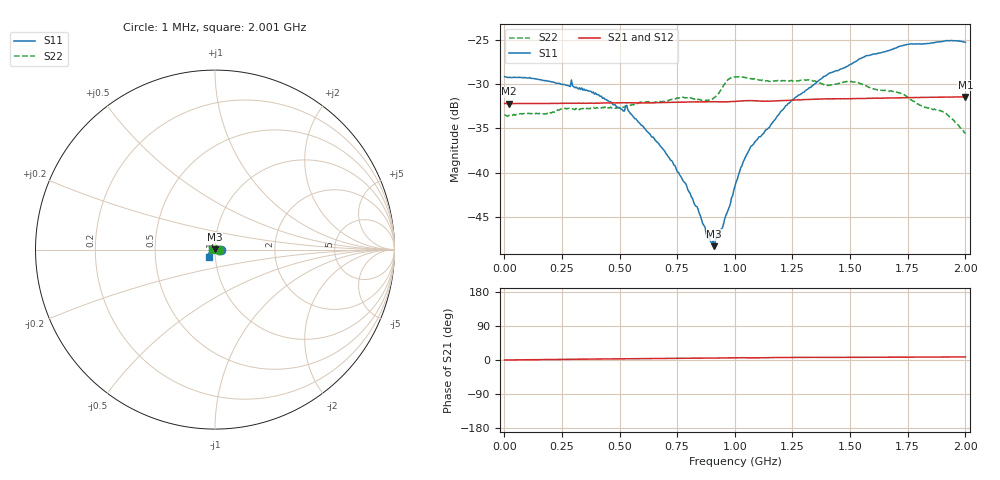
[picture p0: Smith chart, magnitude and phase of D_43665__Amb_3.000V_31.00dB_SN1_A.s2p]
! device id: 43665_
! dir: \\malibu\benchdata\1_engineers\tn_data\43665_75ohm\new\sparar\43665_\amb\3p000v\31p00db
! Serial: 1
! Insertion: A
! Temp: Amb
! VDD: 3.000V
! Attenuation Step: 31.00dB
! IDD: 1.445651e+00mA
! FILE NAME
! DATE 03-27-2009 08:42:13
! CORRECTED  DATA
#  Hz  S  RI  R  75
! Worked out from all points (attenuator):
!   401 points, 1 MHz to 2.001 GHz, reference 75 ohm
!   highest |S21| = -31.44 dB at 2.001 GHz (marker M1); lowest = -32.2 dB at 21 MHz (marker M2)
!   lowest |S11| = -48.3 dB at 911 MHz (marker M3), VSWR 1.01, Z = 74.6 + j0.442 ohm
!   |S11| at or under -10 dB: start of sweep to end of sweep
!   |S22| runs from -35.6 to -29.2 dB; largest |S21 - S12| = 0.00022
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1000000  0.0348 -0.000333  0.0246 4.37e-05  0.0248 -8.65e-05  0.0212 -0.000164
2.1e7  0.0345 0.000212  0.0245 5.04e-05  0.0245 5.75e-05  0.021 0.0012
3.36e8  0.0295 0.00583  0.0246 0.000938  0.0247 0.000944  0.0125 0.0193
5.36e8  0.0212 0.00762  0.0248 0.0014  0.0248 0.00141  0.00159 0.0236
6.71e8  0.0126 0.00719  0.0248 0.00181  0.0248 0.00183  -0.00699 0.024
7.81e8  0.0064 0.00607  0.0249 0.00205  0.0249 0.00209  -0.014 0.0226
8.41e8  0.00266 0.00558  0.025 0.00214  0.025 0.00218  -0.0172 0.0194
8.86e8  -0.00106 0.00431  0.025 0.0022  0.025 0.00222  -0.0197 0.0164
9.11e8  -0.00245 0.00296  0.025 0.00224  0.025 0.00232  -0.0219 0.0149
9.41e8  -0.0043 0.00211  0.025 0.00234  0.025 0.00239  -0.0263 0.0135
9.71e8  -0.00592 0.00164  0.025 0.00246  0.025 0.00251  -0.03 0.0152
1.001e9  -0.00827 0.00141  0.0251 0.00259  0.0251 0.00263  -0.0306 0.0164
1.036e9  -0.0114 0.000566  0.0253 0.00267  0.0253 0.00266  -0.031 0.0154
1.076e9  -0.0142 -0.00141  0.0254 0.00251  0.0254 0.00253  -0.0307 0.0138
1.226e9  -0.023 -0.00702  0.0254 0.00302  0.0254 0.00304  -0.0322 0.00695
1.336e9  -0.0281 -0.0128  0.0257 0.00316  0.0258 0.0032  -0.033 0.00244
1.401e9  -0.0316 -0.0166  0.0259 0.0031  0.0259 0.00317  -0.031 -0.00113
1.496e9  -0.0347 -0.0208  0.0259 0.0032  0.026 0.00324  -0.0324 -0.00398
1.561e9  -0.0374 -0.025  0.026 0.00325  0.0261 0.00329  -0.0306 -0.00598
1.671e9  -0.0389 -0.0299  0.0262 0.00337  0.0262 0.00341  -0.0281 -0.00656
1.906e9  -0.0388 -0.0392  0.0264 0.0037  0.0265 0.00369  -0.0208 -0.00674
2.001e9  -0.0362 -0.0407  0.0265 0.00381  0.0265 0.00377  -0.016 -0.00445
